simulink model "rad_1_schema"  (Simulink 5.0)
settings: Solver=ode45  SolverMode=SingleTasking  StartTime=0.0  StopTime=10.0  RelTol=1e-3
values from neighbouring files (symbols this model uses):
  D = 0    [MWS_1rad_nacitanie.m]    (also in MWS_1rad_udaje.m; MWS_2rad_nacitanie.m; MWS_2rad_udaje.m; MWS_kmitanie_nacitanie.m)
  K = (yx - y0) / (ux - u0)    [MWS_1rad_nacitanie.m]    (also in MWS_1rad_udaje.m; MWS_2rad_nacitanie.m = ( yx - y0 ) / ( ux - u0 ); MWS_2rad_udaje.m = ( yx - y0 ) / ( ux -u0 ); MWS_kmitanie_nacitanie.m = y1 / ( 1 + M ))
  T1 = Tn / f2k    [MWS_2rad_nacitanie.m]    (also in MWS_2rad_udaje.m)

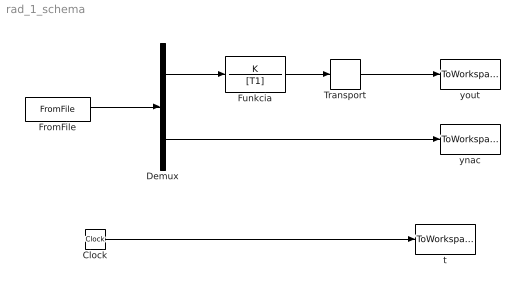
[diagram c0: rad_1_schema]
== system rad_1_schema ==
  Clock : Clock
  Demux : Demux  Outputs=2
  FromFile : FromFile  FileName=data.mat  SampleTime=0
  Funkcia : TransferFcn  Numerator=K  Denominator=[T1]
  Transport : TransportDelay  DelayTime=D
  t : ToWorkspace  VariableName=t  SampleTime=-1  SaveFormat=Array
  ynac : ToWorkspace  VariableName=ynac  SampleTime=-1  SaveFormat=Array
  yout : ToWorkspace  VariableName=yout  SampleTime=-1  SaveFormat=Array
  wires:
  FromFile/1 -> Demux/1
  Demux/1 -> Funkcia/1
  Funkcia/1 -> Transport/1
  Transport/1 -> yout/1
  Demux/2 -> ynac/1
  Clock/1 -> t/1
